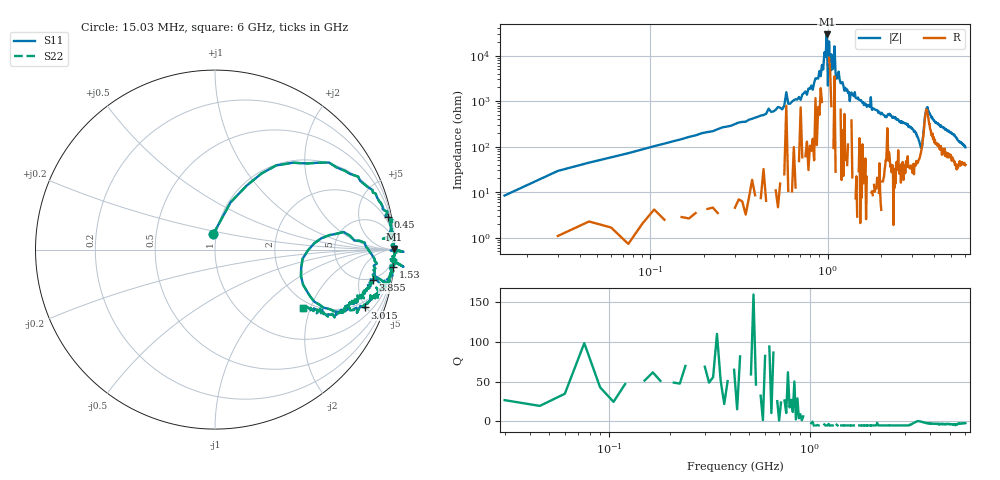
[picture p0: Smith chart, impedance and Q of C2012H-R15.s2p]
!	Network	Analyzer	HP8753E.07.74:	Oct	30	2002	Serial	No.	JP38451487
!	Hewlett-Packard
!	28	Aug	2009	10:44:10
!	Frequency	S11	S21	S12	S22
#	HZ	S	RI	R	50
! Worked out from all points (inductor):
!   400 points, 15.03 MHz to 6 GHz, reference 50 ohm
!   read as one part in series: L = 154 nH near 45.03 MHz
!   highest |Z| = 29.1 kohm at 990 MHz (marker M1)
!   self-resonance near 990 MHz
!   S11 on the Smith chart (normalised r, x): 15.03 MHz: 0.97, +0.16; 450 MHz: 1, +11; 1.53 GHz: 1, -21; 3.015 GHz: 1.53, -4.91; 3.855 GHz: 4.62, -7.93; 6 GHz: 1.79, -1.76
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1.502992e7  -0.0107 0.0847  1.01 -0.0847  1.01 -0.0847  -0.0107 0.0847
3.002985e7  0.0872 0.264  0.913 -0.264  0.913 -0.264  0.0872 0.264
9.002955e7  0.433 0.484  0.567 -0.484  0.567 -0.484  0.433 0.484
4.500278e8  0.963 0.182  0.0367 -0.182  0.0367 -0.182  0.963 0.182
8.250259e8  0.992 0.0554  0.00778 -0.0554  0.00778 -0.0554  0.992 0.0554
9.450253e8  1.01 0.0176  -0.0102 -0.0176  -0.0102 -0.0176  1.01 0.0176
9.90025e8  1 0.00342  -0.0003 -0.00342  -0.0003 -0.00342  1 0.00342
1.005025e9  1.05 -0.0127  -0.0462 0.0127  -0.0462 0.0127  1.05 -0.0127
1.020025e9  0.998 -0.00436  0.00217 0.00436  0.00217 0.00436  0.998 -0.00436
1.035025e9  0.979 -0.00528  0.0209 0.00528  0.0209 0.00528  0.979 -0.00528
1.080025e9  0.999 -0.0173  0.00058 0.0173  0.00058 0.0173  0.999 -0.0173
1.095025e9  0.999 -0.00607  0.0014 0.00607  0.0014 0.00607  0.999 -0.00607
1.125024e9  0.999 -0.0322  0.000824 0.0322  0.000824 0.0322  0.999 -0.0322
1.530022e9  0.991 -0.0952  0.00934 0.0952  0.00934 0.0952  0.991 -0.0952
2.01002e9  0.966 -0.177  0.0338 0.177  0.0338 0.177  0.966 -0.177
3.015015e9  0.834 -0.322  0.166 0.322  0.166 0.322  0.834 -0.322
3.375013e9  0.479 -0.148  0.521 0.148  0.521 0.148  0.479 -0.148
3.615012e9  0.874 -0.0284  0.126 0.0284  0.126 0.0284  0.874 -0.0284
3.855011e9  0.881 -0.168  0.119 0.168  0.119 0.168  0.881 -0.168
4.00501e9  0.866 -0.205  0.134 0.205  0.134 0.205  0.866 -0.205
5.010005e9  0.743 -0.312  0.257 0.312  0.257 0.312  0.743 -0.312
6e9  0.488 -0.323  0.512 0.323  0.512 0.323  0.488 -0.323
